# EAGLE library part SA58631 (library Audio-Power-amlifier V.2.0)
The SA58631 is a one channel audio amplifier in an HVSON8 package. It provides power output of 3 W with an 8 W load at 9 V supply. The internal circuit is comprised of a BTL (Bridge Tied Load) amplifier with a complementary PNP-NPN output stage and standby/mute logic. The SA58631 is housed in an 8-pin HVSON package which has an exposed die attach paddle enabling reduced thermal resistance and increased power dissipation.
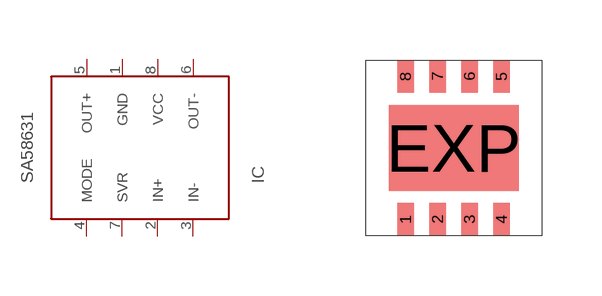
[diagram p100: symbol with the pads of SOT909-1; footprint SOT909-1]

Designator prefix IC

## SA58631HVSON8  [SOT909-1]
1  GND  pwr
2  IN+  in
3  IN-  in
4  MODE
5  OUT+  out
6  OUT-  out
7  SVR
8  VCC  pwr

## Footprint SOT909-1 (pad centres in mm)
smd 0.406 x 0.813: 1 -1.2,-1.79; 2 -0.4,-1.79; 3 0.4,-1.79; 4 1.2,-1.79; 5 1.2,1.79; 6 0.4,1.79; 7 -0.4,1.79; 8 -1.2,1.79
smd 3.25 x 2.15: EXP 0,0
